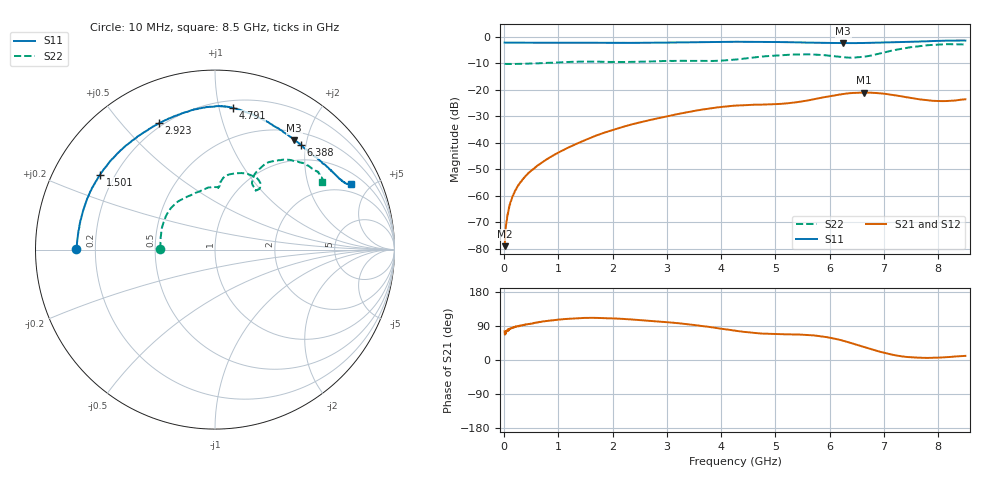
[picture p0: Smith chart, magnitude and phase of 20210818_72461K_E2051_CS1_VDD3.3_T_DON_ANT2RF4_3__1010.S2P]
!Agilent Technologies,E5071C,MY46417908,A.11.23
!Date: Wed Aug 18 14:33:22 2021
!Data & Calibration Information:
!Freq	S11:SOLT2(ON)	S21:SOLT2(ON)	S12:SOLT2(ON)	S22:SOLT2(ON)
!PortZ  Port1:50+j0  Port2:50+j0
!Above PortZ is port z conversion or system Z0 setting when saving the data.
!When reading, reference impedance value at option line is always used.
# Hz S dB R 50
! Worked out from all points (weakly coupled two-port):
!   1601 points, 10 MHz to 8.5 GHz, reference 50 ohm
!   highest |S21| = -21.08 dB at 6.638 GHz (marker M1); lowest = -79.0 dB at 10 MHz (marker M2)
!   lowest |S11| = -2.5 dB at 6.25 GHz (marker M3), VSWR 7.07, Z = 31.8 + j89.1 ohm
!   |S11| at or under -10 dB: nowhere
!   |S22| runs from -10.3 to -2.9 dB; largest |S21 - S12| = 0.00042
!   S11 on the Smith chart (normalised r, x): 10 MHz: 0.13, +0.00; 1.501 GHz: 0.15, +0.29; 2.923 GHz: 0.18, +0.63; 4.791 GHz: 0.26, +1.10; 6.388 GHz: 0.70, +1.90; 8.5 GHz: 1.53, +3.81
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1e7  -2.23 179.7  -78.96 75.6  -80.07 79.6  -10.28 179.6
6.30625e7  -2.27 178.5  -67.26 77.2  -67.03 80.6  -10.30 178.1
1.16125e8  -2.27 177.3  -62.39 83.7  -62.66 82.5  -10.30 176.6
2.063312e8  -2.29 175.2  -57.98 87.6  -58.04 87.5  -10.31 174.2
3.28375e8  -2.29 172.5  -54.28 91.6  -54.20 91.6  -10.26 171.2
4.822562e8  -2.31 169.0  -50.85 95.6  -50.90 95.6  -10.16 167.4
7.634875e8  -2.32 162.7  -46.54 102.5  -46.53 102.6  -9.92 158.7
1.426769e9  -2.33 148.5  -39.55 110.6  -39.58 110.5  -9.43 135.6
1.501056e9  -2.34 146.9  -38.93 111.1  -38.93 111.1  -9.43 133.1
2.17495e9  -2.35 131.8  -34.10 108.6  -34.10 108.6  -9.59 112.8
2.843538e9  -2.29 115.7  -30.75 101.7  -30.75 101.6  -9.30 98.7
2.923131e9  -2.28 113.9  -30.39 100.6  -30.39 100.6  -9.22 97.3
4.255e9  -1.96 89.9  -26.02 77.4  -26.02 77.4  -8.67 86.0
4.790931e9  -1.99 82.9  -25.63 69.4  -25.63 69.5  -7.47 79.9
5.671769e9  -2.28 67.6  -23.76 65.4  -23.77 65.5  -6.73 59.1
6.25015e9  -2.48 54.1  -21.64 50.7  -21.67 50.7  -7.75 54.5
6.388112e9  -2.45 50.8  -21.30 45.0  -21.32 45.0  -7.97 55.4
6.637506e9  -2.40 44.8  -21.08 34.1  -21.12 34.0  -7.55 60.3
7.088538e9  -2.17 35.9  -21.76 15.9  -21.80 15.7  -5.55 60.6
7.592631e9  -1.90 28.7  -23.46 6.3  -23.47 6.2  -3.73 50.2
8.0755e9  -1.57 25.9  -24.30 6.8  -24.28 6.8  -2.94 38.1
8.5e9  -1.50 25.7  -23.62 10.9  -23.64 10.6  -3.01 32.2
